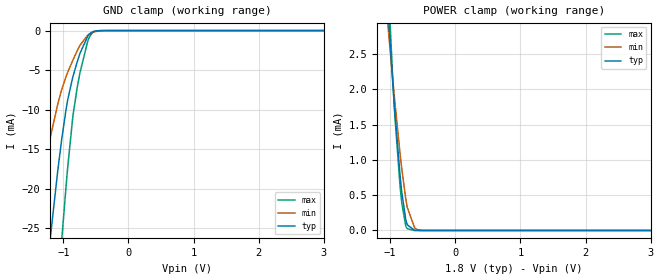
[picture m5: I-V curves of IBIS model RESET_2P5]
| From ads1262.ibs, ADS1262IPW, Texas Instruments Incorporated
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|   Model RESET_2P5
[Model]   RESET_2P5
Model_type   Input
Vinl = 0.50
Vinh = 2.00
|   typ   min   max
|   (nom PVT)   (fast PVT)   (slow PVT)
C_comp   0.211pF   0.208pF   0.222pF
[Model spec]
|subparameter
Vinl   0.50   0.45   0.55
Vinh   2.00   1.80   2.20
[Voltage Range]   1.8   1.65   1.95
[Temperature Range]   27   125   -40
[Power Clamp Reference]   1.8   1.65   1.95
[GND Clamp Reference]   -0   -0   -0
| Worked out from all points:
|   GND clamp passes 1 mA (typ) near -0.64 V on its own axis
|   POWER clamp passes 1 mA (typ) near -0.87 V on its own axis
[GND Clamp]
|   Voltage   I(typ)   I(min)   I(max)
-2.5V     -156.7mA   -92.73mA   -212.9mA
-1.45V    -48.06mA   -25.05mA   -77.61mA
-1.383V   -41.87mA   -21.68mA   -69.07mA
-1.195V   -25.92mA   -13.34mA   -45.96mA
-1.022V   -13.63mA   -7.399mA   -26.31mA
-940mV    -9.107mA   -5.435mA   -18.02mA
-857.5mV  -6.003mA   -3.843mA   -11.18mA
-790mV    -4.058mA   -2.61mA    -7.381mA
-745mV    -2.914mA   -1.868mA   -5.376mA
-625mV    -708uA     -585.1uA   -1.343mA
-542.5mV  -137.4uA   -212.7uA   -223.7uA
4.992V    0A         0A         0A
[POWER Clamp]
|   Voltage   I(typ)   I(min)   I(max)
-2.5V     33.05mA    25.93mA    40.4mA
-1.03V    3.092mA    2.866mA    3.514mA
-1.022V   2.976mA    2.786mA    3.354mA
-962.5mV  2.12mA     2.165mA    2.18mA
-932.5mV  1.733mA    1.868mA    1.683mA
-850mV    801.2uA    1.107mA    651.6uA
-820mV    527.7uA    860.4uA    379.4uA
-760mV    153.4uA    446.1uA    62.07uA
-737.5mV  81.04uA    327uA      24.28uA
-625mV    1.595uA    38.62uA    169.3nA
-512.5mV  3.576nA    1.98uA     0A
4.992V    0A         0A         0A
